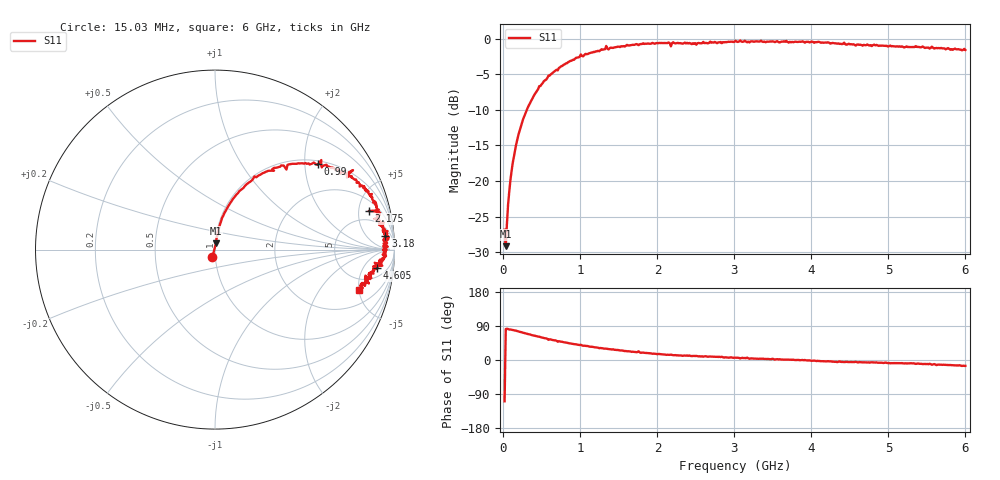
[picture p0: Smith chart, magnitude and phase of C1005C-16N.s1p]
!	Network	Analyzer	HP8753E.07.74:	Oct	30	2002	Serial	No.	JP38451487
!	Hewlett-Packard
!	7	Sep	2009	8:48:05
!	Frequency	S11
#	HZ	S	RI	R	50
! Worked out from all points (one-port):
!   400 points, 15.03 MHz to 6 GHz, reference 50 ohm
!   lowest |S11| = -29.2 dB at 30.03 MHz (marker M1), VSWR 1.07, Z = 50.4 + j3.48 ohm
!   |S11| at or under -10 dB: start of sweep to 303.8 MHz
!   S11 on the Smith chart (normalised r, x): 15.03 MHz: 0.97, -0.08; 990 MHz: 1.09, +2.34; 2.175 GHz: 3.30, +6.42; 3.18 GHz: 11, +18; 4.605 GHz: 9, -10; 6 GHz: 3.46, -4.99
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1.502992e7  -0.0148 -0.043
3.002985e7  0.00503 0.0345
6.00297e7  0.00977 0.0675
1.050295e8  0.0208 0.115
1.650292e8  0.0391 0.176
2.550287e8  0.0839 0.258
4.650277e8  0.22 0.408
7.650262e8  0.43 0.478
9.90025e8  0.575 0.475
1.335023e9  0.769 0.443
1.365023e9  0.735 0.404
1.515022e9  0.789 0.372
1.755021e9  0.827 0.352
1.785021e9  0.866 0.298
1.93502e9  0.895 0.264
2.145019e9  0.913 0.222
2.175019e9  0.856 0.215
2.205019e9  0.92 0.205
2.265019e9  0.911 0.2
2.505017e9  0.89 0.172
2.595017e9  0.937 0.144
3.015015e9  0.961 0.103
3.180014e9  0.949 0.0757
3.765011e9  0.943 0.0144
4.515007e9  0.91 -0.0824
4.605007e9  0.904 -0.104
5.265004e9  0.863 -0.135
6e9  0.801 -0.223
